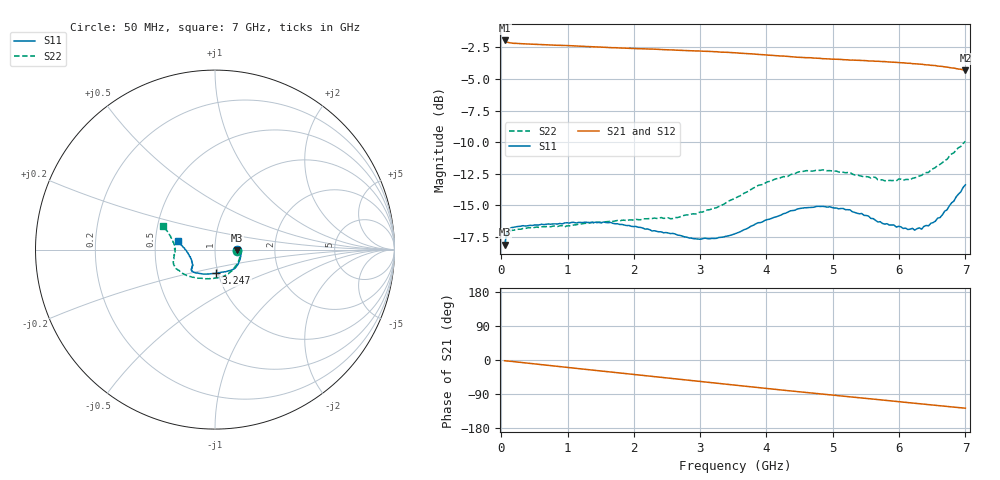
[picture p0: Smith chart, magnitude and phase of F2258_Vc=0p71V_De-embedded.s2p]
! Integrated Device Technology
! Corporate Headquarters
! 6024 Silver Creek Valley Road
! San Jose, CA 95138  USA
! Phone:  1-408-284-8200
! Toll Free:  1-800-223-1366
! Webpage:  http://www.idt.com/
! Timing and RF Division
! 515 Groton Road, Suite 102
! Westford, MA 01886-6024
! Device:  F2258
! Description: Voltage Variable RF Attenuator
! Frequency:  50.0 -  6000.00 MHz
! Package:  3x3 mm Thin QFN Plastic Package: 16 pin
! Ports:  2 RF, 2 DC
!  Pin  1  = NC
!  Pin  2  = NC
!  Pin  3  = RF2  = Port 2
!  Pin  4  = GND
!  Pin  5  = Vdd
!  Pin  6  = NC
!  Pin  7  = VCTRL
!  Pin  8  = NC
!  Pin  9  = GND
!  Pin 10  = RF1  = Port 1
!  Pin 11  = NC
!  Pin 12  = NC
!  Pin 13  = NC
!  Pin 14  = NC
!  Pin 15  = NC
!  Pin 16  = NC
! Vcntrl:  0.710 Volts
! Vdd:  +3.300 Volts
! Current:  1.122 mA
! Data:  The device was measured on a the F2258 evaluation board which has
!  individual transmission lines to the RF pins.  Data was collected
!  using a calibrated network analyzer.  The evaluation board was
!  de-embedded using a TRL calibration technique.
!  The reference plane is the edge of the package pin.
! Misc:  SN 10
!  Action Tracker AT0285
! Date Measured:  2014-12-10
! Date:  2016-01-13  MJV
! Note:
!  Integrated Device Technology supplies this data as a sample of measured
!  data at the package pin for this product.  Your particular data for this
!  product may vary.
!  Data was taken at 25 degrees C.
!  Integrated Device Technology reserves the right to change this data at anytime.
!Freq_(GHz)  S11M_(dB)  S11P_(deg)  S21M_(dB)  S21P_(deg)  S12M_(dB)  S12P_(deg)  S22M_(dB)  S22P_(deg)
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# GHz S dB R 50
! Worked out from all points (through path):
!   201 points, 50 MHz to 7 GHz, reference 50 ohm
!   highest |S21| = -1.95 dB at 50 MHz (marker M1); lowest = -4.3 dB at 7 GHz (marker M2)
!   group delay of S21, straight-line fit = 50.4 ps
!   lowest |S11| = -18.1 dB at 50 MHz (marker M3), VSWR 1.28, Z = 64.1 - j0.48 ohm
!   |S11| at or under -10 dB: start of sweep to end of sweep
!   |S22| runs from -18.2 to -9.9 dB; largest |S21 - S12| = 0.0015
!   S11 on the Smith chart (normalised r, x): 50 MHz: 1.28, -0.01; 3.247 GHz: 0.98, -0.26; 7 GHz: 0.65, +0.07
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0.05  -18.13 -1.7  -1.95 -2.0  -1.94 -2.0  -18.25 -2.6
0.08475  -17.18 -2.9  -2.08 -2.5  -2.06 -2.5  -17.35 -3.9
0.15425  -16.77 -4.8  -2.15 -3.7  -2.15 -3.7  -17.00 -6.8
0.745  -16.51 -22.6  -2.31 -14.9  -2.30 -14.9  -16.71 -30.3
1.2315  -16.38 -36.2  -2.42 -24.0  -2.42 -24.0  -16.47 -48.8
1.6485  -16.36 -44.6  -2.52 -31.6  -2.52 -31.5  -16.26 -61.6
2.37825  -17.11 -58.2  -2.66 -44.8  -2.65 -44.8  -16.03 -81.5
2.58675  -17.24 -63.4  -2.70 -48.6  -2.69 -48.6  -16.06 -88.0
2.8995  -17.65 -73.4  -2.77 -54.4  -2.76 -54.4  -15.68 -98.8
3.247  -17.62 -87.7  -2.84 -61.0  -2.84 -61.0  -15.19 -112.6
3.525  -17.26 -100.5  -2.93 -66.2  -2.92 -66.2  -14.46 -123.9
4.0115  -16.14 -120.4  -3.11 -75.3  -3.10 -75.3  -13.15 -141.0
4.359  -15.45 -129.6  -3.23 -81.6  -3.22 -81.6  -12.59 -150.9
4.7065  -15.17 -135.6  -3.34 -87.7  -3.35 -87.7  -12.29 -157.8
5.2625  -15.38 -140.9  -3.51 -97.3  -3.52 -97.3  -12.42 -167.0
5.85325  -16.58 -147.8  -3.65 -107.5  -3.65 -107.5  -13.04 -178.2
6.166  -16.90 -155.7  -3.76 -113.0  -3.76 -113.0  -13.01 175.0
6.2355  -16.98 -159.3  -3.80 -114.1  -3.80 -114.2  -12.83 172.9
6.444  -16.64 -168.8  -3.89 -117.9  -3.90 -117.9  -12.41 168.0
6.61775  -15.98 -178.2  -3.99 -120.9  -4.00 -120.9  -11.77 163.3
6.722  -15.37 177.3  -4.06 -122.7  -4.07 -122.7  -11.37 160.6
7  -13.39 166.7  -4.31 -127.2  -4.32 -127.2  -9.94 155.1
